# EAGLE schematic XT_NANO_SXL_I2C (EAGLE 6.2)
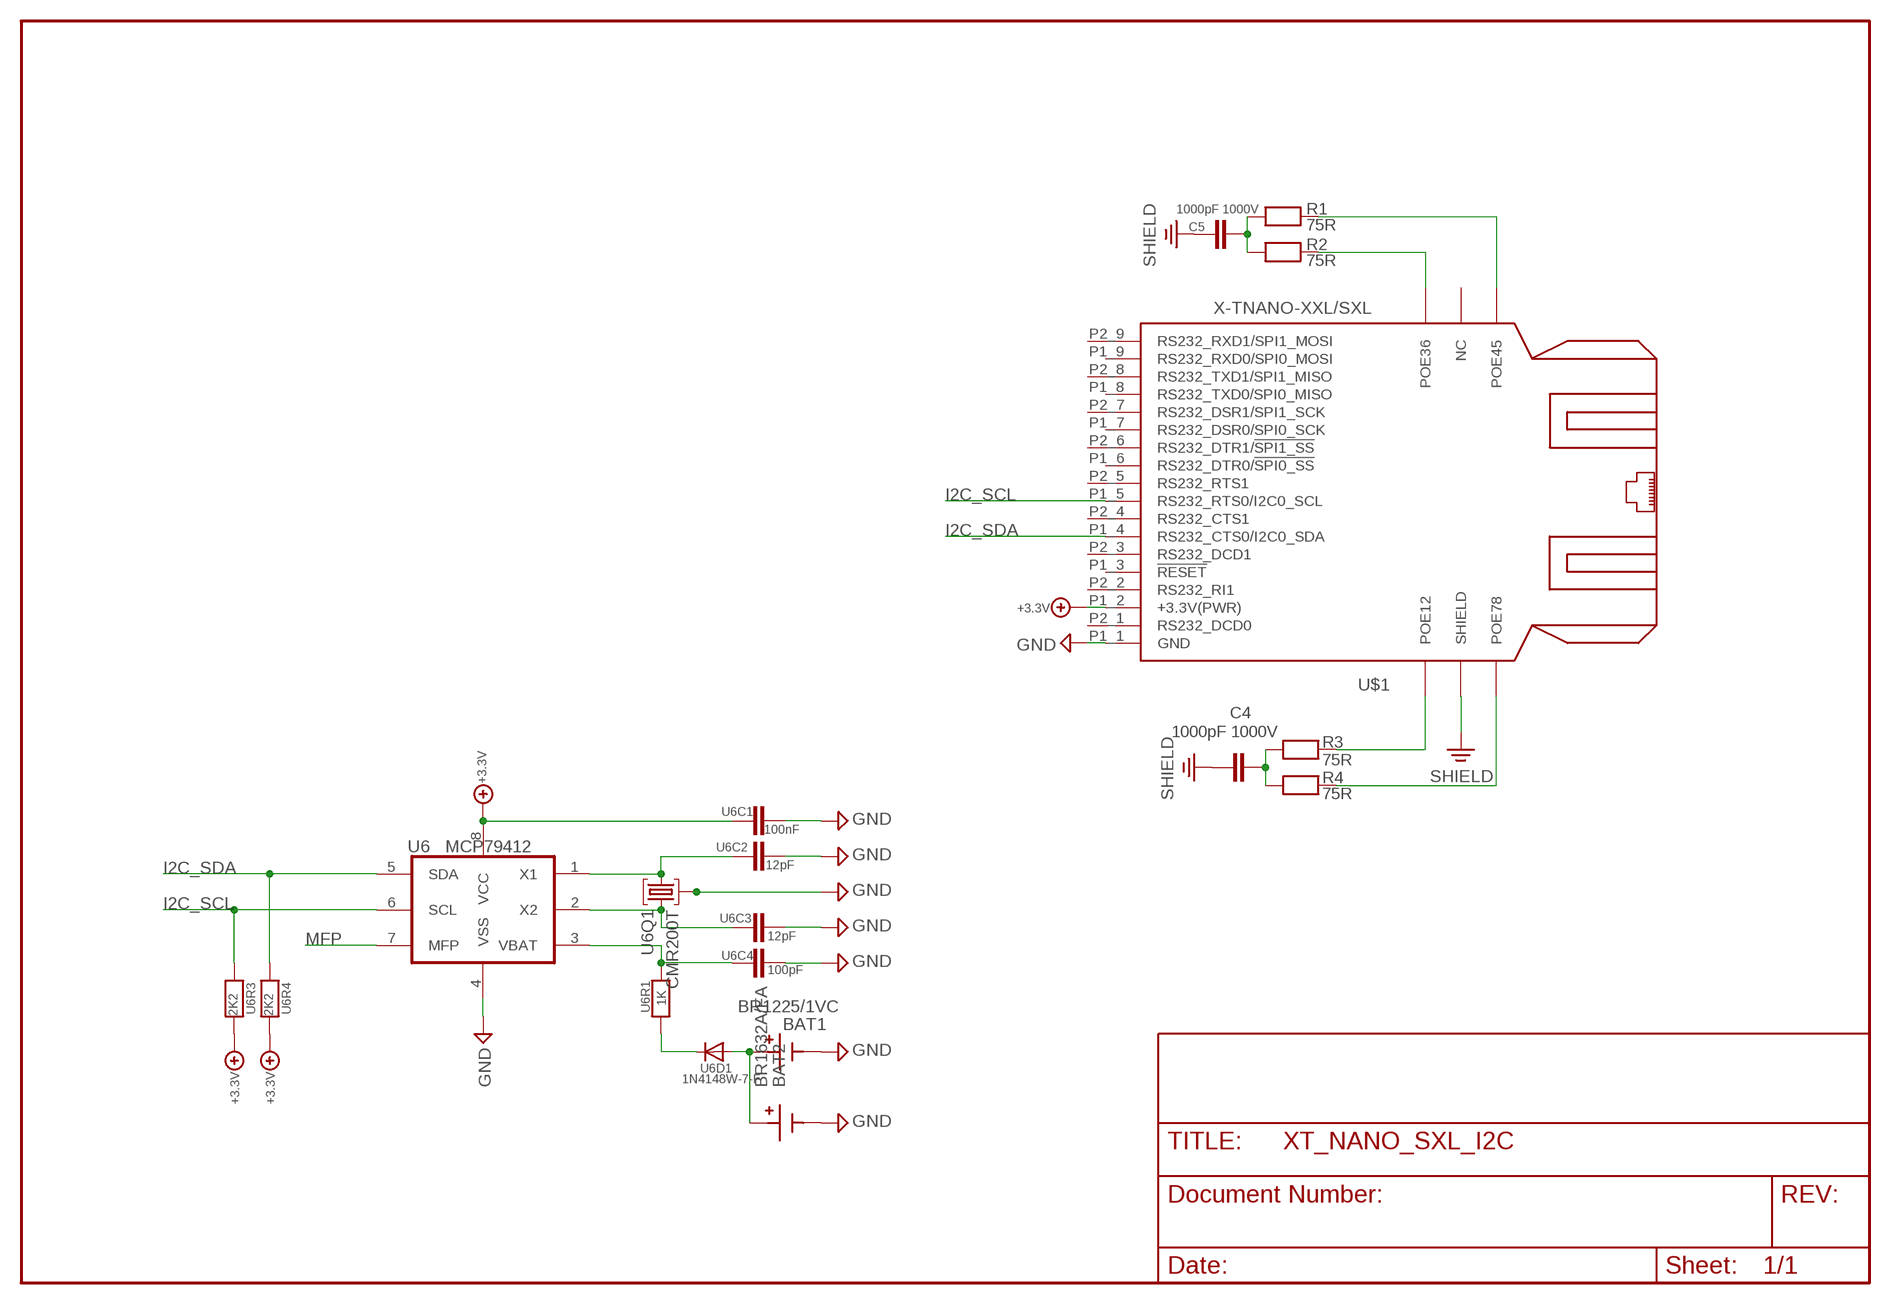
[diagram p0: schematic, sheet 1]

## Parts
BAT1  BR1225/1VC  [BR1225VC]
BAT2  BR1632A/FA  [BR1632A/FA]
C4  1000pF 1000V  CHIP-C-1210  [SMD-1210]
C5  1000pF 1000V  CHIP-C-1210  [SMD-1210]
R1  75R  CHIP-R-0603  [SMD-0603]
R2  75R  CHIP-R-0603  [SMD-0603]
R3  75R  CHIP-R-0603  [SMD-0603]
R4  75R  CHIP-R-0603  [SMD-0603]
U6  MCP79412  [SO-8]
U6C1  100nF  CHIP-C-VTS0402  [R0402_VTS@1]
U6C2  12pF  CHIP-C-VTS0402  [R0402_VTS@1]
U6C3  12pF  CHIP-C-VTS0402  [R0402_VTS@1]
U6C4  100pF  CHIP-C-VTS0402  [R0402_VTS@1]
U6D1  1N4148W-7-F  DIODE-SOD123  [SOD123]
U6Q1  CMR200T  [CMR200T]
U6R1  1K  CHIP-R-VTS04020402_VTS  [R0402_VTS]
U6R3  2K2  CHIP-R-VTS04020402_VTS  [R0402_VTS]
U6R4  2K2  CHIP-R-VTS04020402_VTS  [R0402_VTS]
U$1  X-TNANO-XXL/SXL  [XT-NANO-XXL/SXL]

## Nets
+3.3V: U6.8(VCC) U6C1.1 U6R3.2 U6R4.2 U$1.P1_2(+3.3V(PWR))
GND: BAT1.2 BAT2.P- U6.4(VSS) U6C1.2 U6C2.1 U6C3.1 U6C4.2 U6Q1.EXP U$1.P1_1(GND)
I2C_SCL: U6.6(SCL) U6R3.1 U$1.P1_5(RS232_RTS0/I2C0_SCL)
I2C_SDA: U6.5(SDA) U6R4.1 U$1.P1_4(RS232_CTS0/I2C0_SDA)
MFP: U6.7(MFP)
N$1: C5.1 R1.1 R2.1
N$2: C4.2 R3.1 R4.1
N$4: R2.2 U$1.POE36
N$6: R1.2 U$1.POE45
N$20: R3.2 U$1.POE12
N$21: R4.2 U$1.POE78
N$30: U6.2(X2) U6C3.2 U6Q1.2
N$34: U6.1(X1) U6C2.2 U6Q1.1
N$36: U6.3(VBAT) U6C4.1 U6R1.2
N$45: U6D1.C U6R1.1
N$46: BAT1.1 BAT2.P+ U6D1.A
SHIELD: C4.1 C5.2 U$1.SHIELD
Unconnected: U$1.FLASH(NC) U$1.P1_3(!RESET) U$1.P1_6(RS232_DTR0/!SPI0_SS!) U$1.P1_7(RS232_DSR0/SPI0_SCK) U$1.P1_8(RS232_TXD0/SPI0_MISO) U$1.P1_9(RS232_RXD0/SPI0_MOSI) U$1.P2_1(RS232_DCD0) U$1.P2_2(RS232_RI1) U$1.P2_3(RS232_DCD1) U$1.P2_4(RS232_CTS1) U$1.P2_5(RS232_RTS1) U$1.P2_6(RS232_DTR1/!SPI1_SS!) U$1.P2_7(RS232_DSR1/SPI1_SCK) U$1.P2_8(RS232_TXD1/SPI1_MISO) U$1.P2_9(RS232_RXD1/SPI1_MOSI)

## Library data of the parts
BAT1 = ak-nord:BR1225/1VC: Panasonic BR-1225/VCN Lithium Battery 3V 48mAh 12,5mm
BAT2 = ak-nord:BR1632A/FA: Panasonic BR1632A/FA Lithium Battery 3V 120mAh d=16mm
C4 C5 = XTMACRO:CHIP-C-?: Chip capacitance
R1-R4 = XTMACRO:CHIP-R-?: Chip resistors
U6 = ak-nord:MCP79412: I2C Real-Time Clock/Calendar with EEPROM, SRAM, Unique ID and Battery Switchover
U6C1-U6C4 = mea-lib:CHIP-C-?: Chip capacitance
U6D1 = diode:DIODE-: DIODE
U6Q1 = ak-nord:CMR200T
U6R1 U6R3 U6R4 = mea-lib:CHIP-R-?: Chip resistors
U$1 = ak-devices:X-TNANO-XXL/SXL: AK-NORD XT-NANO-XXL/SXL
